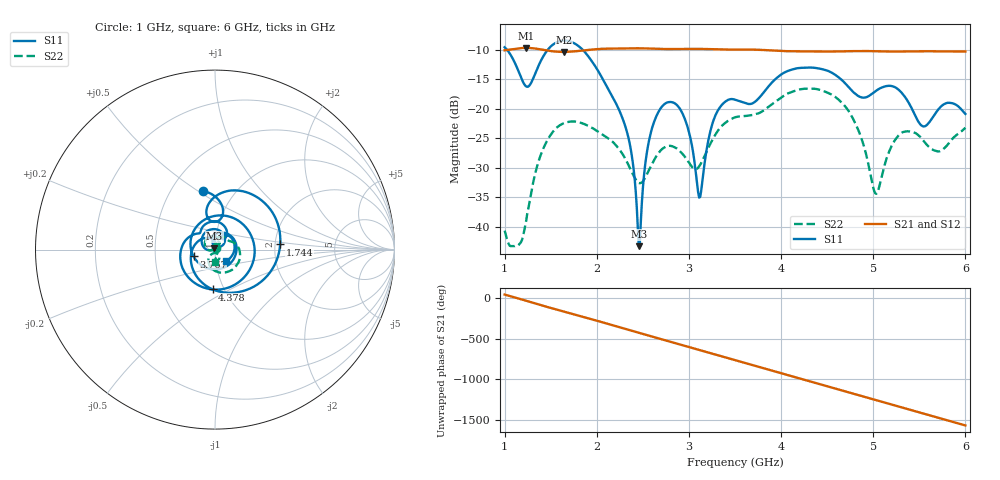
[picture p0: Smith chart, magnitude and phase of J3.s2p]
!Agilent Technologies,E8364B,MY43040528,A.07.50.67
!Agilent E8364B: A.07.50.67
!Date: Sunday, March 01, 2026 18:18:38
!Correction: S11(Full 2 Port(1,2))
!S21(Full 2 Port(1,2))
!S12(Full 2 Port(1,2))
!S22(Full 2 Port(1,2))
!S2P File: Measurements: S11, S21, S12, S22:
# Hz S  dB  R 50
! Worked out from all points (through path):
!   451 points, 1 GHz to 6 GHz, reference 50 ohm
!   highest |S21| = -9.64 dB at 1.233 GHz (marker M1); lowest = -10.3 dB at 1.644 GHz (marker M2)
!   group delay of S21, straight-line fit = 897 ps
!   lowest |S11| = -43.3 dB at 2.456 GHz (marker M3), VSWR 1.01, Z = 49.7 + j0.619 ohm
!   |S11| at or under -10 dB: 1.028 GHz to 1.466 GHz (438.1 MHz wide, 35.1 % of centre); 1.85 GHz to end of sweep
!   |S22| runs from -43.3 to -16.6 dB; largest |S21 - S12| = 0.0015
!   S11 on the Smith chart (normalised r, x): 1 GHz: 0.71, +0.52; 1.744 GHz: 2.13, +0.14; 3.767 GHz: 0.78, -0.06; 4.378 GHz: 0.88, -0.41; 6 GHz: 1.13, -0.15
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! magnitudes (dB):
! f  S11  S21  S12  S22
! 1 GHz  -9.5  -10.0  -10.1  -40.6
! 1.233 GHz  -16.2  -9.6  -9.7  -39.0
! 1.4 GHz  -11.6  -9.9  -9.9  -27.5
! 1.644 GHz  -8.4  -10.3  -10.4  -22.4
! 1.744 GHz  -8.8  -10.2  -10.3  -22.1
! 1.844 GHz  -9.9  -10.1  -10.1  -22.4
! 2.311 GHz  -23.0  -9.7  -9.8  -28.5
! 2.456 GHz  -43.3  -9.7  -9.7  -32.5
! 2.556 GHz  -26.3  -9.7  -9.8  -30.7
! 2.667 GHz  -20.6  -9.8  -9.8  -27.6
! 2.922 GHz  -20.5  -9.8  -9.9  -27.5
! 3.111 GHz  -35.0  -9.8  -9.8  -29.7
! 3.278 GHz  -21.4  -9.9  -9.9  -24.6
! 3.5 GHz  -18.4  -9.9  -10.0  -21.4
! 3.767 GHz  -18.0  -10.0  -10.0  -20.7
! 4.344 GHz  -13.0  -10.3  -10.3  -16.6
! 4.378 GHz  -13.0  -10.3  -10.3  -16.6
! 4.756 GHz  -16.7  -10.2  -10.2  -20.9
! 5.022 GHz  -17.0  -10.2  -10.2  -34.3
! 5.167 GHz  -16.1  -10.3  -10.3  -27.4
! 5.533 GHz  -22.9  -10.2  -10.2  -25.2
! 6 GHz  -20.8  -10.3  -10.3  -23.2
